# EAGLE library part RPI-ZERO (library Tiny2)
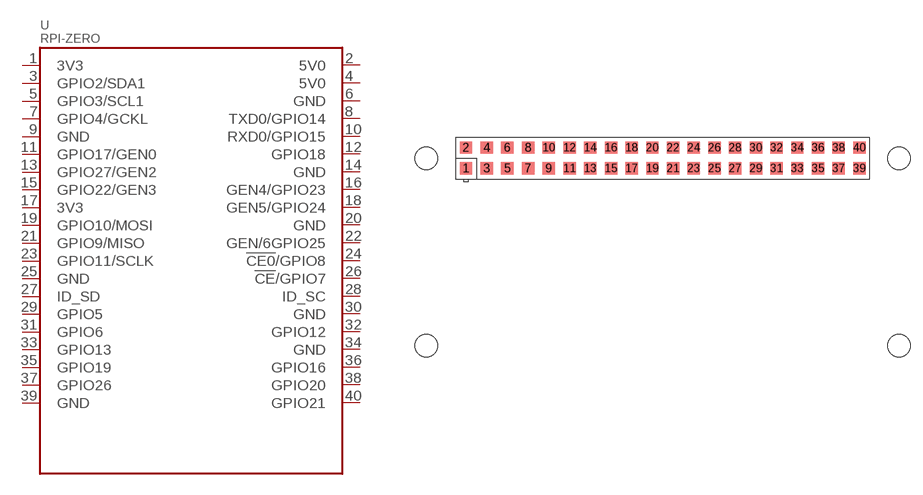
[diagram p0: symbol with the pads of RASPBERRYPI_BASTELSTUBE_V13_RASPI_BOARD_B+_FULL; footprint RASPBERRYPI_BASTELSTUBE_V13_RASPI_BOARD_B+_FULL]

Designator prefix -

## RPI-ZERO  [RASPBERRYPI_BASTELSTUBE_V13_RASPI_BOARD_B+_FULL]
1  3V3  sup
2  5V0  sup
3  GPIO2/SDA1
4  5V0  sup
5  GPIO3/SCL1
6  GND  sup
7  GPIO4/GCKL
8  TXD0/GPIO14
9  GND  sup
10  RXD0/GPIO15
11  GPIO17/GEN0
12  GPIO18
13  GPIO27/GEN2
14  GND  sup
15  GPIO22/GEN3
16  GEN4/GPIO23
17  3V3  sup
18  GEN5/GPIO24
19  GPIO10/MOSI
20  GND  sup
21  GPIO9/MISO
22  GEN/6GPIO25
23  GPIO11/SCLK
24  !CE0!/GPIO8
25  GND  sup
26  !CE!/GPIO7
27  ID_SD
28  ID_SC
29  GPIO5
30  GND  sup
31  GPIO6
32  GPIO12
33  GPIO13
34  GND  sup
35  GPIO19
36  GPIO16
37  GPIO26
38  GPIO20
39  GND  sup
40  GPIO21

## Footprint RASPBERRYPI_BASTELSTUBE_V13_RASPI_BOARD_B+_FULL (pad centres in mm)
Raspberry Pi board model B+, full outline with position of big connectors & drill holes
smd 1.524 x 1.524: 1 8.382,25.273; 2 8.382,27.813; 3 10.922,25.273; 4 10.922,27.813; 5 13.462,25.273; 6 13.462,27.813; 7 16.002,25.273; 8 16.002,27.813; 9 18.542,25.273; 10 18.542,27.813; 11 21.082,25.273; 12 21.082,27.813; 13 23.622,25.273; 14 23.622,27.813; 15 26.162,25.273; 16 26.162,27.813; 17 28.702,25.273; 18 28.702,27.813; 19 31.242,25.273; 20 31.242,27.813; 21 33.782,25.273; 22 33.782,27.813; 23 36.322,25.273; 24 36.322,27.813; 25 38.862,25.273; 26 38.862,27.813; 27 41.402,25.273; 28 41.402,27.813; 29 43.942,25.273; 30 43.942,27.813; 31 46.482,25.273; 32 46.482,27.813; 33 49.022,25.273; 34 49.022,27.813; 35 51.562,25.273; 36 51.562,27.813; 37 54.102,25.273; 38 54.102,27.813; 39 56.642,25.273; 40 56.642,27.813
hole 2.75 at 3.5,3.5
hole 2.75 at 3.5,26.5
hole 2.75 at 61.5,3.5
hole 2.75 at 61.5,26.5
